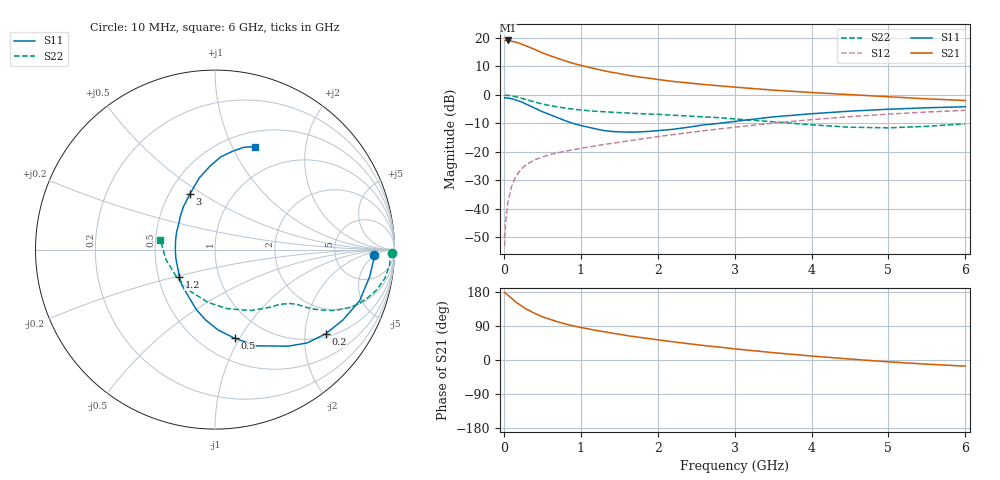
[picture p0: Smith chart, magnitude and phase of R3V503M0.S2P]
! SIEMENS Small Signal Semiconductors
! BFR181
! Si NPN RF Bipolar Junction Transistor in SOT23
! VCE = 0.5 V  IC = 3 mA
! Common Emitter S-Parameters:  May  1996
# GHz  S  MA  R  50
!  f  S11  S21  S12  S22
! GHz  MAG  ANG  MAG  ANG  MAG  ANG  MAG  ANG
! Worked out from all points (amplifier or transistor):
!   36 points, 10 MHz to 6 GHz, reference 50 ohm
!   highest |S21| = 19.1 dB at 50 MHz (marker M1)
!   |S21| within 3 dB of that: start of sweep to 387.7 MHz
!   unconditionally stable (mu >= 1): 1.052 GHz to 4.14 GHz
!   at 250 MHz: K = 0.35, MSG = 21.5 dB, |S12| = -25.4 dB
!   at 1.4 GHz: K = 1.12, MAG = 10.4 dB, |S12| = -17.1 dB
!   at 6 GHz: K = 0.97, MSG = 1.7 dB, |S12| = -5.5 dB
!   S11 on the Smith chart (normalised r, x): 10 MHz: 15, -4; 200 MHz: 1.09, -2.55; 500 MHz: 0.72, -0.96; 1.2 GHz: 0.64, -0.21; 3 GHz: 0.63, +0.45; 6 GHz: 0.67, +1.23
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0.01  0.8837 -1.9  8.922 178.5  0.0022 90.0  0.9843 -1.0
0.02  0.8852 -3.9  8.958 176.3  0.0051 88.9  0.9765 -2.0
0.05  0.8749 -9.9  8.994 171.3  0.0124 84.1  0.977 -4.9
0.1  0.8547 -19.5  8.72 163.0  0.0244 78.5  0.9599 -9.6
0.15  0.8137 -28.8  8.437 153.8  0.0355 73.4  0.9282 -14.0
0.2  0.7746 -37.3  8.063 146.7  0.0448 69.6  0.891 -17.6
0.3  0.6762 -52.7  7.107 133.5  0.0605 62.8  0.8198 -23.1
0.4  0.5847 -66.5  6.27 123.2  0.0722 57.9  0.7478 -27.0
0.5  0.5068 -77.4  5.46 114.2  0.0809 55.0  0.6886 -29.3
0.6  0.4482 -87.8  4.863 107.3  0.0892 53.1  0.6472 -30.9
0.7  0.3962 -97.5  4.365 100.8  0.0957 52.2  0.612 -32.0
0.8  0.3504 -107.2  3.927 95.1  0.1022 51.6  0.5836 -32.8
0.9  0.3137 -115.4  3.569 90.1  0.1085 51.6  0.5592 -33.4
1.1  0.2695 -133.5  3.053 82.0  0.1209 51.7  0.5265 -35.0
1.2  0.251 -142.1  2.84 78.0  0.1271 51.9  0.5137 -35.8
1.6  0.2211 -176.4  2.22 64.5  0.1542 52.6  0.4797 -39.5
2.2  0.2481 144.4  1.716 48.0  0.2 52.3  0.4376 -47.6
3  0.341 114.1  1.363 29.4  0.2696 48.4  0.3772 -63.3
3.5  0.4091 102.3  1.208 19.4  0.3185 44.4  0.3365 -78.2
4.5  0.5166 86.6  1.007 2.5  0.4131 33.7  0.2698 -120.4
5.5  0.5919 74.3  0.848 -11.0  0.4982 21.1  0.2798 -169.0
6  0.6164 68.7  0.794 -16.2  0.5337 14.2  0.309 169.7
